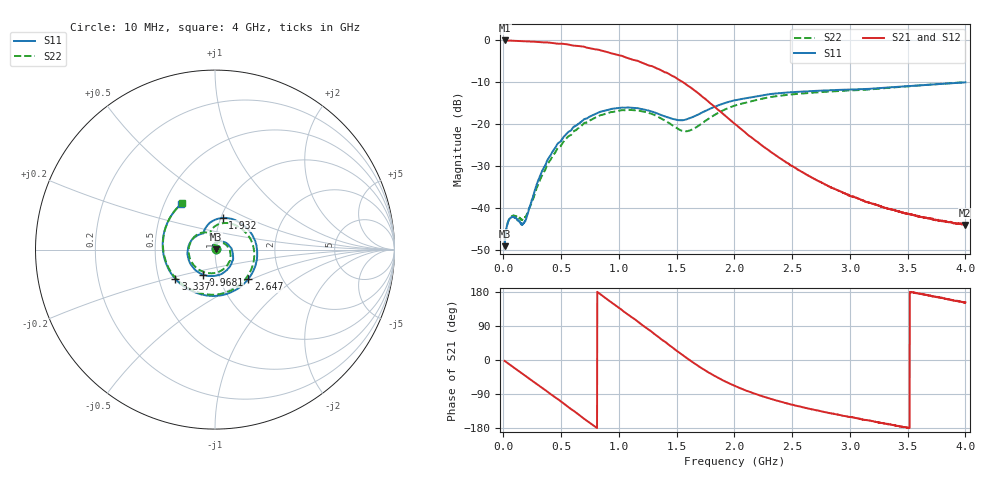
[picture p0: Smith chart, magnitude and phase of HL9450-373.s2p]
! 7/13/2020 7:55:56 AM
! H:\PRODUCTION_DATA\9450\10015\HL9450_10009_938MHZ_.S2P
! CHANNEL.1
! TR.MEASUREMENT
! CORRECTED.DATA
# GHZ S RI R 50.0
! FREQ.GHZ  S11RE  S11IM  S21RE  S21IM  S12RE  S12IM  S22RE  S22IM
!; PortSelection: Port_12
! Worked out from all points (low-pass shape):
!   2000 points, 10 MHz to 4 GHz, reference 50 ohm
!   highest |S21| = -0.03 dB at 10 MHz (marker M1); lowest = -44.0 dB at 3.998 GHz (marker M2)
!   |S21| within 3 dB of the highest: start of sweep to 925.9 MHz
!   lowest |S11| = -49.1 dB at 10 MHz (marker M3), VSWR 1.01, Z = 50.3 + j0.191 ohm
!   |S11| at or under -10 dB: start of sweep to end of sweep
!   |S22| runs from -49.0 to -10.0 dB; largest |S21 - S12| = 0.0079
!   S11 on the Smith chart (normalised r, x): 10 MHz: 1.01, +0.00; 968.1 MHz: 0.84, -0.24; 1.932 GHz: 1.02, +0.37; 2.647 GHz: 1.36, -0.48; 3.337 GHz: 0.61, -0.22; 4 GHz: 0.61, +0.34
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0.01  0.00297 0.0019  0.996 -0.0399  0.9971 -0.0406  0.003 0.00191
0.06389195  0.00761 -0.000736  0.9616 -0.2442  0.9613 -0.2447  0.00775 -0.00112
0.1836518  -0.00449 -0.00514  0.7444 -0.6347  0.7438 -0.6354  -0.00443 -0.00619
0.3652876  -0.00404 0.0331  0.1636 -0.9329  0.1633 -0.9323  -0.00453 0.029
0.5109955  0.0531 0.0417  -0.3463 -0.8429  -0.3462 -0.8431  0.048 0.0352
0.6766633  0.1008 -0.0393  -0.7302 -0.4297  -0.7307 -0.4287  0.0863 -0.0427
0.8203752  0.0481 -0.1282  -0.7736 0.0268  -0.7703 0.0274  0.0281 -0.1207
0.968079  -0.0674 -0.139  -0.559 0.3933  -0.5565 0.3916  -0.083 -0.1158
1.157699  -0.1529 -0.0289  -0.1248 0.5588  -0.1268 0.5525  -0.1464 0.00656
1.341331  -0.1136 0.0688  0.2215 0.3986  0.2228 0.3954  -0.0796 0.0925
1.588834  -0.0621 0.0964  0.2924 0.0242  0.2926 0.024  -0.0247 0.0789
1.932146  0.0434 0.1764  0.0642 -0.1039  0.0639 -0.1043  0.0418 0.147
2.005998  0.0866 0.1728  0.0369 -0.0935  0.0364 -0.0938  0.0802 0.1468
2.341326  0.2294 0.0299  -0.0114 -0.0428  -0.0116 -0.0427  0.2128 0.019
2.646713  0.1851 -0.1646  -0.015 -0.0189  -0.0151 -0.0188  0.1691 -0.1649
2.670665  0.1746 -0.1769  -0.0149 -0.0177  -0.0149 -0.0177  0.1585 -0.1767
2.988029  -0.0163 -0.2587  -0.0125 -0.0073  -0.0124 -0.00724  -0.0284 -0.2507
3.335333  -0.2194 -0.1647  -0.00968 -0.0018  -0.00972 -0.0018  -0.2247 -0.1525
3.337329  -0.2205 -0.1638  -0.00964 -0.00177  -0.00967 -0.00183  -0.2254 -0.1517
3.662676  -0.2907 0.0442  -0.00763 0.00112  -0.00756 0.00121  -0.289 0.0568
3.998004  -0.192 0.2508  -0.00547 0.00315  -0.00557 0.0031  -0.1831 0.2596
4  -0.1908 0.2518  -0.0057 0.00297  -0.00555 0.00311  -0.182 0.2605
